(*
-------------------------------------------------------------------------------------------------------

This function copies the data from an array of BYTE to an array of BOOL.

Parameter
 INPUT:
 - pSourceBoolArr [INPUT] - pointer to the source array of BOOL
 - nSizeBoolSrc [INPUT] - size of the source array in BYTE
 - pDestByteArr [INPUT] - pointer to the destination array of BYTE
 - nSizeBytes [INPUT] - size of the destination array in BYTE
 
Return
 [BOOL]:
 
 - TRUE => function succeeded
 - FALSE => function failed (destination array is not big enough or at least one address pointer is zero)
 
-------------------------------------------------------------------------------------------------------
*)

FUNCTION F_ByteArrToBoolArr : BOOL
VAR_INPUT
	pSrcByteArr		: POINTER TO BYTE;		// pointer to the source array of BYTE 
	nSizeByteSrc	: UDINT;                // size of the source array in BYTE
	pDestBoolArr	: POINTER TO BOOL;      // pointer to the destination array of BOOL
	nSizeBoolDest	: UDINT;                // size of the destination array in BYTE
	
END_VAR
VAR
	idx				: UDINT;				// index FOR-loop
	nSampeCnt		: UDINT;                // total sample counter
END_VAR

// input validation 
IF pSrcByteArr <> 0 AND pDestBoolArr <> 0 THEN
	// check size of the destination
	IF nSizeBoolDest >= nSizeByteSRC * 8 THEN
		// copy data in FOR-loop
		FOR idx := 0 TO nSizeByteSRC - 1 DO
			pDestBoolArr[nSampeCnt] := pSrcByteArr[idx].0;
			nSampeCnt := nSampeCnt + 1;
			pDestBoolArr[nSampeCnt] := pSrcByteArr[idx].1;
			nSampeCnt := nSampeCnt + 1;
			pDestBoolArr[nSampeCnt] := pSrcByteArr[idx].2;
			nSampeCnt := nSampeCnt + 1;
			pDestBoolArr[nSampeCnt] := pSrcByteArr[idx].3;
			nSampeCnt := nSampeCnt + 1;
			pDestBoolArr[nSampeCnt] := pSrcByteArr[idx].4;
			nSampeCnt := nSampeCnt + 1;
			pDestBoolArr[nSampeCnt] := pSrcByteArr[idx].5;
			nSampeCnt := nSampeCnt + 1;
			pDestBoolArr[nSampeCnt] := pSrcByteArr[idx].6;
			nSampeCnt := nSampeCnt + 1;
			pDestBoolArr[nSampeCnt] := pSrcByteArr[idx].7;
			nSampeCnt := nSampeCnt + 1;
		END_FOR
		F_ByteArrToBoolArr := TRUE;		// function succeeded
	ELSE
		F_ByteArrToBoolArr := FALSE;	// function failed because the destination array is not big enough
	END_IF
ELSE
	F_ByteArrToBoolArr := FALSE;		// funtion failed bacause at least one address pointer is zero
END_IF

END_FUNCTION
